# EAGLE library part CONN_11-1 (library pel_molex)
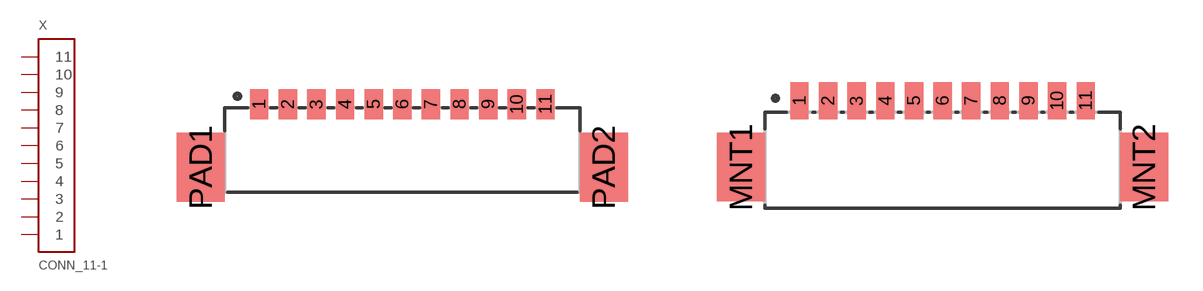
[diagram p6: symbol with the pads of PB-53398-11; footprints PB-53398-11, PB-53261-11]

Designator prefix X

## CONN_11-1-53398  [PB-53398-11]
1  1
2  2
3  3
4  4
5  5
6  6
7  7
8  8
9  9
10  10
11  11

## CONN_11-1-53261  [PB-53261-11]
Pads as for PB-53398-11

## CONN_11-1-53047  [PB-53047-11]
Pads as for PB-53398-11

## Footprint PB-53398-11 (pad centres in mm)
smd 0.8 x 1.3: 1 -6.25,1.25; 2 -5,1.25; 3 -3.75,1.25; 4 -2.5,1.25; 5 -1.25,1.25; 6 0,1.25; 7 1.25,1.25; 8 2.5,1.25; 9 3.75,1.25; 10 5,1.25; 11 6.25,1.25
smd 2.1 x 3: PAD1 -8.8,-1.5; PAD2 8.8,-1.5

## Footprint PB-53261-11 (pad centres in mm)
smd 0.8 x 1.6: 1 -6.25,1.1; 2 -5,1.1; 3 -3.75,1.1; 4 -2.5,1.1; 5 -1.25,1.1; 6 0,1.1; 7 1.25,1.1; 8 2.5,1.1; 9 3.75,1.1; 10 5,1.1; 11 6.25,1.1
smd 2.1 x 3: MNT1 -8.8,-1.8; MNT2 8.8,-1.8

## Footprint PB-53047-11 (pad centres in mm)
drill 0.5: 1 -6.25,0; 2 -5,0; 3 -3.75,0; 4 -2.5,0; 5 -1.25,0; 6 0,0; 7 1.25,0; 8 2.5,0; 9 3.75,0; 10 5,0; 11 6.25,0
